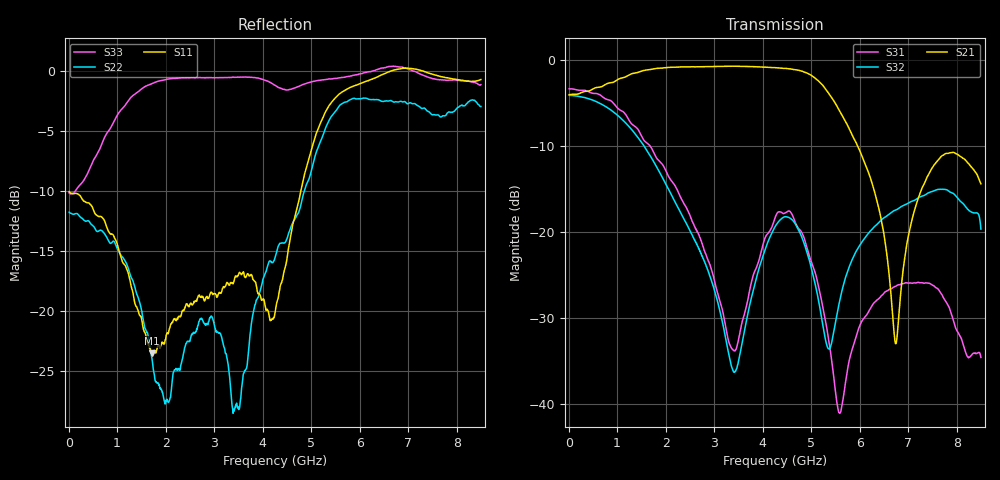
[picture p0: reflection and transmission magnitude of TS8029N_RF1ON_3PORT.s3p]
!Created with skrf (http://scikit-rf.org).
# GHz S RI R 50.0
!freq ReS11 ImS11 ReS12 ImS12 ReS13 ImS13
! ReS21 ImS21 ReS22 ImS22 ReS23 ImS23
! ReS31 ImS31 ReS32 ImS32 ReS33 ImS33
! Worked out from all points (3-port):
!   1601 points, 10 MHz to 8.5 GHz, reference 50 ohm
!   strongest paths, dB at 10 MHz, 2.132 GHz, 4.255 GHz, 6.378 GHz, 8.5 GHz:
!     S21: -4.0, -0.8, -0.9, -16.8, -14.4
!     S32: -4.1, -15.8, -19.4, -19.0, -19.6
!     S31: -3.3, -14.1, -18.3, -27.8, -34.6
!   lowest |S11| = -23.6 dB at 1.724 GHz (marker M1), VSWR 1.14, Z = 56.7 + j2.17 ohm
!   |S11| at or under -10 dB: start of sweep to 4.788 GHz
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0.01  -0.3139 0.00532  0.6303 0.00018  0.6823 -0.00944
      0.6301 0.000126  -0.2575 0.00393  0.6254 -0.00934
      0.6822 -0.00953  0.6256 -0.00937  -0.3096 0.0131
1.723919  0.0636 0.0191  0.7087 -0.5342  -0.1749 -0.2467
          0.7084 -0.534  -0.00154 0.0617  -0.1679 -0.2052
          -0.1747 -0.2464  -0.1681 -0.2055  0.6758 -0.5727
3.406  -0.1132 -0.0677  -0.0727 -0.9202  -0.0129 -0.016
       -0.0722 -0.9201  -0.0209 0.0323  0.00066 0.0153
       -0.0129 -0.016  0.000677 0.0154  -0.6311 -0.6971
4.255  0.00394 0.0981  -0.5751 -0.6993  -0.0592 -0.1059
       -0.5753 -0.6988  -0.1396 -0.0906  0.0669 -0.0841
       -0.0592 -0.1057  0.067 -0.084  -0.7622 0.4201
5.082775  0.4996 0.1755  -0.7829 -0.0476  -0.0355 0.0461
          -0.7839 -0.0471  -0.4258 0.1192  -0.037 -0.0336
          -0.0355 0.0461  -0.0369 -0.0337  0.9052 0.0685
5.586869  0.8014 -0.053  -0.4508 0.2314  0.00884 -0.000469
          -0.4509 0.2312  -0.4281 0.5749  0.0224 -0.0328
          0.00884 -0.000475  0.0224 -0.0328  0.7641 -0.5392
6.738325  0.7381 -0.6912  -0.0224 0.00205  -0.0388 -0.0291
          -0.0225 0.00202  0.5795 0.4662  -0.0333 -0.1306
          -0.0387 -0.0291  -0.0334 -0.1303  0.3913 -0.9678
7.125681  0.6167 -0.8099  -0.0747 -0.1088  -0.0483 -0.0151
          -0.0746 -0.1093  0.7304 0.0275  -0.0894 -0.1247
          -0.0485 -0.0151  -0.0895 -0.1241  0.44 -0.8925
7.815494  0.5041 -0.7876  -0.2846 -0.0432  -0.0274 0.0263
          -0.2834 -0.044  -0.1699 -0.6472  -0.1745 -0.000451
          -0.0273 0.0261  -0.175 0.000148  0.2865 -0.867
8.5  0.5734 -0.7195  -0.1478 0.1214  0.00499 0.018
     -0.1475 0.1216  -0.5929 0.3907  0.0157 0.103
     0.005 0.018  0.0156 0.103  0.0331 -0.8749
